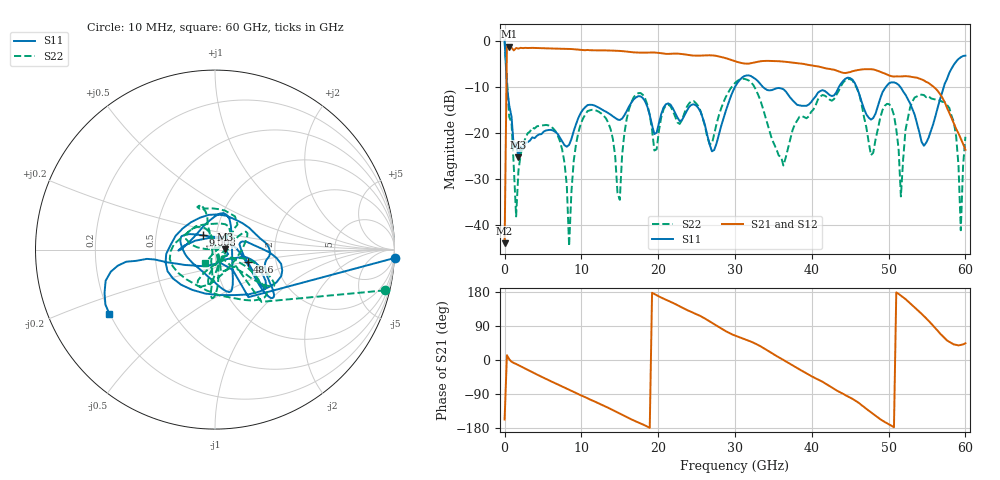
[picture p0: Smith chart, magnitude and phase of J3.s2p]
!Keysight Technologies,N5227A,US51270214,A.10.65.11
!Date: Thursday, October 15, 2020 07:42:45
!Correction: S11(Full 2 Port(1,2))
!S21(Full 2 Port(1,2))
!S12(Full 2 Port(1,2))
!S22(Full 2 Port(1,2))
!S2P File: Measurements: S11, S21, S12, S22:
# Hz S  dB  R 50
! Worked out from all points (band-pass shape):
!   201 points, 10 MHz to 60 GHz, reference 50 ohm
!   highest |S21| = -1.27 dB at 609.9 MHz (marker M1); lowest = -44.0 dB at 10 MHz (marker M2)
!   |S21| within 3 dB of the highest: 289.6 MHz to 29.69 GHz (29.4 GHz wide, 196 % of centre)
!   lowest |S11| = -25.3 dB at 1.81 GHz (marker M3), VSWR 1.11, Z = 55.7 + j0.119 ohm
!   |S11| at or under -10 dB: 324.8 MHz to 30.01 GHz (29.69 GHz wide, 196 % of centre); 33.61 GHz to 43.55 GHz (9.933 GHz wide, 25.7 % of centre); 51.51 GHz to 57.19 GHz (5.683 GHz wide, 10.5 % of centre)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
!   |S22| runs from -44.6 to -0.2 dB; largest |S21 - S12| = 0.13
!   S11 on the Smith chart (normalised r, x): 10 MHz: -6, -43; 9.008 GHz: 0.86, +0.14; 48.6 GHz: 1.43, -0.21; 60 GHz: 0.20, -0.27
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1e7  0.06 -2.6  -43.98 -157.0  -46.75 -165.7  -0.22 -13.5
3.0995e8  -9.79 -54.9  -1.38 12.7  -2.07 20.6  -8.18 -48.3
6.099e8  -14.00 -51.7  -1.27 2.0  -1.22 7.3  -16.55 -38.3
1.50975e9  -22.20 -19.0  -1.58 -10.5  -1.40 -9.3  -38.15 -26.8
1.8097e9  -25.30 1.1  -1.70 -13.6  -1.56 -12.8  -28.21 33.2
6.6089e9  -19.79 49.0  -1.71 -61.4  -1.69 -61.4  -19.57 26.5
8.4086e9  -22.60 104.1  -1.78 -78.5  -1.78 -78.7  -44.60 81.2
9.0085e9  -19.61 130.2  -1.84 -84.5  -1.84 -84.5  -26.06 176.6
1.02083e10  -14.96 151.7  -2.03 -95.6  -2.01 -95.7  -16.92 167.3
1.50075e10  -17.21 -127.5  -2.22 -141.2  -2.22 -141.2  -34.54 -62.5
1.68072e10  -12.75 -77.5  -2.53 -159.4  -2.54 -159.4  -12.31 -88.8
2.010665e10  -17.84 44.2  -2.65 167.7  -2.66 167.7  -19.48 21.1
3.0005e10  -10.02 -38.6  -4.46 64.4  -4.48 64.3  -9.18 -26.6
3.630395e10  -10.53 3.4  -4.50 0.2  -4.54 0.3  -27.09 -25.0
4.02033e10  -12.68 160.7  -5.42 -45.1  -5.43 -45.4  -14.95 147.0
4.86019e10  -14.21 -20.8  -6.55 -151.8  -6.51 -151.8  -19.20 -98.3
5.010165e10  -9.17 -38.1  -7.56 -170.6  -7.56 -170.2  -13.80 -99.7
5.16014e10  -10.19 -28.9  -7.76 170.0  -7.74 169.8  -33.81 -131.9
5.310115e10  -14.83 -13.8  -7.88 144.1  -7.89 144.4  -13.18 103.9
5.790035e10  -7.00 -171.9  -15.65 48.0  -15.61 47.7  -14.58 47.9
5.94001e10  -3.59 -158.6  -21.26 39.7  -21.25 40.0  -41.15 -35.8
6e10  -3.24 -148.9  -23.68 44.1  -23.67 44.6  -20.86 -126.1
